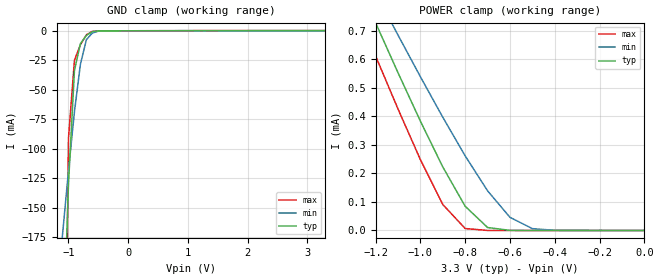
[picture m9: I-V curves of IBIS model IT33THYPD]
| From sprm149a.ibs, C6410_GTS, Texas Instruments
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[Model]   IT33THYPD
Model_type   Input
Polarity   Non-Inverting
| signals   A, Y
Vinl = 0.8V
Vinh = 2.0V
|   typ   min   max
C_comp   1.5797p   1.5046p   1.7659p
|   typ   min   max
[Temperature Range]   25   -40   125
|   typ   min   max
[Voltage Range]   3.30V   3.00V   3.60V
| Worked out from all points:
|   GND clamp passes 1 mA (typ) near -0.61 V on its own axis
|   POWER clamp passes 1 mA (typ) near -1.35 V on its own axis
[GND_clamp]
|   Voltage   I(typ)   I(min)   I(max)
-3.3V     -4.396A    -1.514A    -19.03A
-1.1V     -280.6mA   -173.2mA   -561.3mA
-1V       -130.3mA   -118.8mA   -91.31mA
-900mV    -33.67mA   -68.7mA    -25.02mA
-800mV    -10.88mA   -28.37mA   -11.81mA
-700mV    -3.947mA   -7.562mA   -3.415mA
-600mV    -797.1uA   -1.866mA   -451.8uA
-500mV    -113uA     -355.1uA   -87.59uA
-400mV    -39.93uA   -61.49uA   -56.44uA
3.3V      100.9uA    52.19uA    177.6uA
[POWER_clamp]
|   Voltage   I(typ)   I(min)   I(max)
-3.3V     4.599mA    4.102mA    4.747mA
-1.3V     905.1uA    983.5uA    800.7uA
-1.2V     727.5uA    833.2uA    611.3uA
-1.1V     552.9uA    684.6uA    425.8uA
-1V       383.1uA    538.7uA    248.1uA
-900mV    222.6uA    396.7uA    91.01uA
-800mV    84.79uA    261.3uA    6.786uA
-700mV    10.3uA     138.9uA    73.9nA
-600mV    329.8nA    46.05uA    977pA
-500mV    8.438nA    6.46uA     266.4pA
-400mV    444.1pA    466.6nA    310.9pA
0V        1pA        1pA        1pA
